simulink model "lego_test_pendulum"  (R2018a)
settings: Solver=VariableStepAuto  StartTime=0.0  StopTime=3  RelTol=1e-3
model workspace: external: MATLAB File (data not in the file)
undefined symbols (not defined in the file): cm, deg, kg, m, mm, N, rad, s, smiData, X, Y, Z
libraries: sm_lib x60, nesl_utility x3, simulink_extras x2
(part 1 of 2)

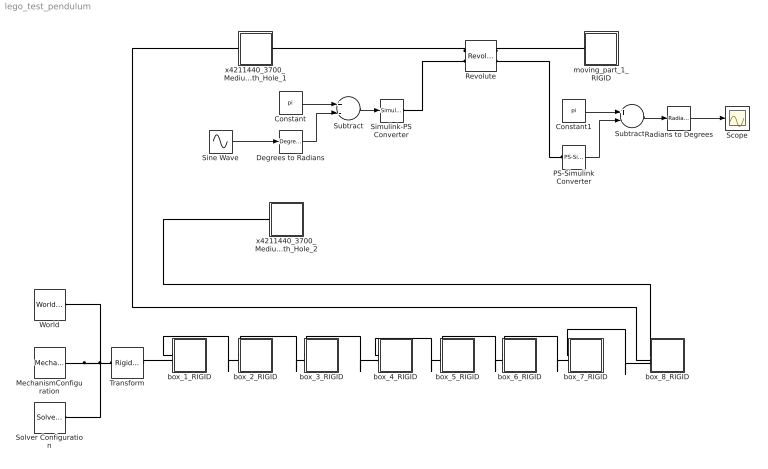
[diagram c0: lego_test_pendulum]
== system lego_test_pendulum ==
  Constant : Constant  Value=pi
  Constant1 : Constant  Value=pi
  Degrees to Radians : simulink_extras/Transformations/Degrees to Radians
  MechanismConfiguration : sm_lib/Utilities/Mechanism Configuration  UniformGravity=Constant  GravityVector=[0 -9.80665 0]  GravityUnits=m/s^2  LinearizationDelta=0.001
  PS-Simulink Converter : nesl_utility/PS-Simulink Converter  PhysicalDomain=network_engine_domain  SubClassName=ps_output  LeftPortType=input  RightPortType=output  PseudoPeriodic=off  Frequencies=[]  Unit=rad  AffineConversion=off
  Radians to Degrees : simulink_extras/Transformations/Radians to Degrees
  Revolute : sm_lib/Joints/Revolute Joint  SenseConstraintForce=off  SenseConstraintForceX=off  SenseConstraintForceY=off  SenseConstraintForceZ=off  SenseConstraintTorque=off  SenseConstraintTorqueX=off  SenseConstraintTorqueY=off  SenseConstraintTorqueZ=off  SenseTotalForce=off  SenseTotalForceX=off  SenseTotalForceY=off  SenseTotalForceZ=off  SenseTotalTorque=off  SenseTotalTorqueX=off  SenseTotalTorqueY=off  SenseTotalTorqueZ=off  CompositeWrenchDir=FollowerOnBase  CompositeWrenchFrame=BaseFrame  EquilibriumPosition=0  EquilibriumPositionUnits=rad  SpringStiffness=0  SpringStiffnessUnits=N*m/rad  DampingCoefficient=0  DampingCoefficientUnits=N*m/(rad/s)  TorqueActuationMode=ComputedTorque  MotionActuationMode=InputMotion  SensePosition=on  SenseVelocity=off  SenseAcceleration=off  SenseTorqueForce=off  PositionTargetSpecify=on  PositionTargetPriority=Low  PositionTargetValue=pi  PositionTargetValueUnits=rad  VelocityTargetSpecify=off  VelocityTargetPriority=High  VelocityTargetValue=0  VelocityTargetValueUnits=deg/s
  Scope : Scope
  Simulink-PS Converter : nesl_utility/Simulink-PS Converter  PhysicalDomain=network_engine_domain  SubClassName=ps_input  LeftPortType=input  RightPortType=output  PseudoPeriodic=off  Frequencies=[]  NoiseDistribution=none  NoiseParameters=[]  Unit=rad  AffineConversion=off  FilteringAndDerivatives=filter  SimscapeFilterOrder=2  InputFilterTimeConstant=0.001  UdotUserProvided=0
  Sine Wave : Sin  Amplitude=30  Frequency=2*pi  SampleTime=0
  Solver Configuration : nesl_utility/Solver Configuration  PhysicalDomain=network_engine_domain  SubClassName=solver  LeftPortType=input  RightPortType=generic  Tones=[]  Harmonics=[]  SimulateNoise=off  Profile=off  UseLocalSampling=off  EnableSwitchedLinearOptims=on  FrequencyDomain=off  UseCCode=off  RelTol=0.001  AbsTol=1e-06  MinStep=1e-09  ToWorkspace=off  RevertToSquareIcSolve=off  NumHomotopyIterations=100  PhasorMode=off  PhasorModeNumHarmonics=1  DoDC=off  ResidualTolerance=1e-09  UseLocalSolver=off  LocalSolverChoice=NE_BACKWARD_EULER_ADVANCER  LocalSolverSampleTime=0.001  DoFixedCost=off  MaxNonlinIter=3  MaxModeIter=2  LinearAlgebra=Sparse  EquationFormulation=NE_TIME_EF  DelaysMemoryBudget=1024  AutomaticFiltering=on  FilteringTimeConstant=0.001
  Subtract : Sum  Inputs=+-
  Subtract1 : Sum  Inputs=+-
  Transform : sm_lib/Frames and Transforms/Rigid Transform  TranslationMethod=Cartesian  TranslationStandardOffset=0  TranslationLengthUnit=mm  TranslationStandardAxis=+Z  TranslationCartesianOffset=smiData.RigidTransform(26).translation  TranslationROffset=0  TranslationROffsetUnits=m  TranslationZOffset=0  TranslationZOffsetUnits=m  TranslationThetaOffset=0  TranslationThetaOffsetUnits=deg  RotationMethod=ArbitraryAxis  RotationAngleUnits=rad  RotationStandardAxis=+Z  RotationAngle=smiData.RigidTransform(26).angle  RotationArbitraryAxis=smiData.RigidTransform(26).axis  FollAlignAxisA=+X  BaseAlignAxisA=+Y  FollAlignAxisB=+Y  BaseAlignAxisB=+Z  RotationSequenceAxes=FollowerAxes  RotationSequence=XYX  RotationSequenceAngles=[0 0 0]  RotationSequenceAnglesUnits=deg  RotationMatrix=[1 0 0; 0 1 0; 0 0 1]
  World : sm_lib/Frames and Transforms/World Frame
  box_1_RIGID : Subsystem
  box_2_RIGID : Subsystem
  box_3_RIGID : Subsystem
  box_4_RIGID : Subsystem
  box_5_RIGID : Subsystem
  box_6_RIGID : Subsystem
  box_7_RIGID : Subsystem
  box_8_RIGID : Subsystem
  moving_part_1_RIGID : Subsystem
  x4211440_3700_Medium_Stone_Grey_Technic_Brick_1_x_2_with_Hole_1 : Subsystem
  x4211440_3700_Medium_Stone_Grey_Technic_Brick_1_x_2_with_Hole_2 : Subsystem
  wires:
  Radians to Degrees/1 -> Scope/1
  Constant/1 -> Subtract/1
  Subtract/1 -> Simulink-PS Converter/1
  Constant1/1 -> Subtract1/1
  PS-Simulink Converter/1 -> Subtract1/2
  Subtract1/1 -> Radians to Degrees/1
  Degrees to Radians/1 -> Subtract/2
  Sine Wave/1 -> Degrees to Radians/1
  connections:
  Transform/LConn1 -- MechanismConfiguration/RConn1 -- Solver Configuration/RConn1 -- World/RConn1
  Revolute/LConn1 -- x4211440_3700_Medium_Stone_Grey_Technic_Brick_1_x_2_with_Hole_1/RConn1
  box_8_RIGID/LConn2 -- x4211440_3700_Medium_Stone_Grey_Technic_Brick_1_x_2_with_Hole_1/LConn1
  box_8_RIGID/LConn1 -- x4211440_3700_Medium_Stone_Grey_Technic_Brick_1_x_2_with_Hole_2/LConn1
  Transform/RConn1 -- box_1_RIGID/LConn2
  Revolute/RConn1 -- moving_part_1_RIGID/LConn1
  box_1_RIGID/LConn1 -- box_2_RIGID/LConn2
  box_2_RIGID/LConn1 -- box_3_RIGID/LConn2
  box_3_RIGID/LConn1 -- box_4_RIGID/LConn2
  box_4_RIGID/LConn1 -- box_5_RIGID/LConn2
  box_5_RIGID/LConn1 -- box_6_RIGID/LConn2
  box_6_RIGID/LConn1 -- box_7_RIGID/LConn2
  box_7_RIGID/LConn1 -- box_8_RIGID/LConn3
  PS-Simulink Converter/LConn1 -- Revolute/RConn2
  Simulink-PS Converter/RConn1 -- Revolute/LConn2

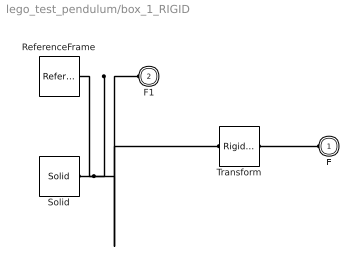
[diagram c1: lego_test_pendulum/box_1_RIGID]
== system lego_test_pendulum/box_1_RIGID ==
  ReferenceFrame : sm_lib/Frames and Transforms/Reference Frame
  Solid : sm_lib/Body Elements/Solid  InertiaType=Custom  Mass=smiData.Solid(1).mass  MassUnits=kg  CenterOfMass=smiData.Solid(1).CoM  CenterOfMassUnits=mm  MomentsOfInertia=smiData.Solid(1).MoI  MomentsOfInertiaUnits=kg*mm^2  ProductsOfInertia=smiData.Solid(1).PoI  ProductsOfInertiaUnits=kg*mm^2  DensityBased=on  Density=1000  DensityUnits=kg/m^3  DoExposeReferenceFrame=on  SerializedFrames=<Frames/>  GraphicType=FromGeometry  MarkerShape=Sphere  MarkerSize=10  GraphicVisPropType=SimpleVisualProperties  GraphicDiffuseColor=smiData.Solid(1).color  GraphicSpecularColor=[0.5 0.5 0.5 1.0]  GraphicAmbientColor=[0.15 0.15 0.15 1.0]  GraphicEmissiveColor=[0.0 0.0 0.0 1.0]  GraphicShininess=75  GraphicOpacity=smiData.Solid(1).opacity  GeometryShape=FromFile  RectangleSize=[1 1]  RectangleSizeUnits=m  BrickDimensions=[1 1 1]  BrickDimensionUnits=m  CylinderRadius=1  CylinderRadiusUnits=m  CylinderLength=1  CylinderLengthUnits=m  SphereRadius=1  SphereRadiusUnits=m  EllipsoidRadii=[1 1 1]  EllipsoidRadiiUnits=m  ExtrusionCrossSection=[1 1; -1 1; -1 -1; 1 -1]  ExtrusionCrossSectionUnits=m  ExtrusionLength=1  ExtrusionLengthUnits=m  PolygonNumSides=3  PolygonOuterRadius=1  PolygonOuterRadiusUnits=m  ExtGeomFileType=STEP  ExtGeomFileName=box_Predeterminado_sldprt.STEP  ExtGeomFileUnits=m  RevolutionCrossSection=[1 1; 1 -1; 2 -1; 2 1]  RevolutionCrossSectionUnits=m  RevolutionExtent=Full  RevolutionAngle=180  RevolutionAngleUnits=deg
  Transform : sm_lib/Frames and Transforms/Rigid Transform  TranslationMethod=Cartesian  TranslationStandardOffset=0  TranslationLengthUnit=mm  TranslationStandardAxis=+Z  TranslationCartesianOffset=smiData.RigidTransform(3).translation  TranslationROffset=0  TranslationROffsetUnits=m  TranslationZOffset=0  TranslationZOffsetUnits=m  TranslationThetaOffset=0  TranslationThetaOffsetUnits=deg  RotationMethod=ArbitraryAxis  RotationAngleUnits=rad  RotationStandardAxis=+Z  RotationAngle=smiData.RigidTransform(3).angle  RotationArbitraryAxis=smiData.RigidTransform(3).axis  FollAlignAxisA=+X  BaseAlignAxisA=+Y  FollAlignAxisB=+Y  BaseAlignAxisB=+Z  RotationSequenceAxes=FollowerAxes  RotationSequence=XYX  RotationSequenceAngles=[0 0 0]  RotationSequenceAnglesUnits=deg  RotationMatrix=[1 0 0; 0 1 0; 0 0 1]
  F : PMIOPort  Side=Left
  F1 : PMIOPort  Port=2  Side=Left
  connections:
  Solid/RConn1 -- ReferenceFrame/RConn1 -- Transform/LConn1 -- F1/RConn1
  Transform/RConn1 -- F/RConn1

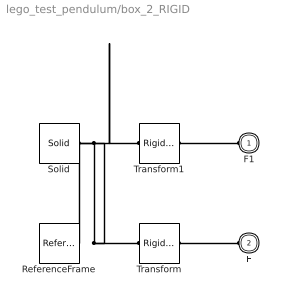
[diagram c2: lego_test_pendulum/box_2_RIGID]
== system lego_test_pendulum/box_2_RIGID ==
  ReferenceFrame : sm_lib/Frames and Transforms/Reference Frame
  Solid : sm_lib/Body Elements/Solid  InertiaType=Custom  Mass=smiData.Solid(1).mass  MassUnits=kg  CenterOfMass=smiData.Solid(1).CoM  CenterOfMassUnits=mm  MomentsOfInertia=smiData.Solid(1).MoI  MomentsOfInertiaUnits=kg*mm^2  ProductsOfInertia=smiData.Solid(1).PoI  ProductsOfInertiaUnits=kg*mm^2  DensityBased=on  Density=1000  DensityUnits=kg/m^3  DoExposeReferenceFrame=on  SerializedFrames=<Frames/>  GraphicType=FromGeometry  MarkerShape=Sphere  MarkerSize=10  GraphicVisPropType=SimpleVisualProperties  GraphicDiffuseColor=smiData.Solid(1).color  GraphicSpecularColor=[0.5 0.5 0.5 1.0]  GraphicAmbientColor=[0.15 0.15 0.15 1.0]  GraphicEmissiveColor=[0.0 0.0 0.0 1.0]  GraphicShininess=75  GraphicOpacity=smiData.Solid(1).opacity  GeometryShape=FromFile  RectangleSize=[1 1]  RectangleSizeUnits=m  BrickDimensions=[1 1 1]  BrickDimensionUnits=m  CylinderRadius=1  CylinderRadiusUnits=m  CylinderLength=1  CylinderLengthUnits=m  SphereRadius=1  SphereRadiusUnits=m  EllipsoidRadii=[1 1 1]  EllipsoidRadiiUnits=m  ExtrusionCrossSection=[1 1; -1 1; -1 -1; 1 -1]  ExtrusionCrossSectionUnits=m  ExtrusionLength=1  ExtrusionLengthUnits=m  PolygonNumSides=3  PolygonOuterRadius=1  PolygonOuterRadiusUnits=m  ExtGeomFileType=STEP  ExtGeomFileName=box_Predeterminado_sldprt.STEP  ExtGeomFileUnits=m  RevolutionCrossSection=[1 1; 1 -1; 2 -1; 2 1]  RevolutionCrossSectionUnits=m  RevolutionExtent=Full  RevolutionAngle=180  RevolutionAngleUnits=deg
  Transform : sm_lib/Frames and Transforms/Rigid Transform  TranslationMethod=Cartesian  TranslationStandardOffset=0  TranslationLengthUnit=mm  TranslationStandardAxis=+Z  TranslationCartesianOffset=smiData.RigidTransform(4).translation  TranslationROffset=0  TranslationROffsetUnits=m  TranslationZOffset=0  TranslationZOffsetUnits=m  TranslationThetaOffset=0  TranslationThetaOffsetUnits=deg  RotationMethod=ArbitraryAxis  RotationAngleUnits=rad  RotationStandardAxis=+Z  RotationAngle=smiData.RigidTransform(4).angle  RotationArbitraryAxis=smiData.RigidTransform(4).axis  FollAlignAxisA=+X  BaseAlignAxisA=+Y  FollAlignAxisB=+Y  BaseAlignAxisB=+Z  RotationSequenceAxes=FollowerAxes  RotationSequence=XYX  RotationSequenceAngles=[0 0 0]  RotationSequenceAnglesUnits=deg  RotationMatrix=[1 0 0; 0 1 0; 0 0 1]
  Transform1 : sm_lib/Frames and Transforms/Rigid Transform  TranslationMethod=Cartesian  TranslationStandardOffset=0  TranslationLengthUnit=mm  TranslationStandardAxis=+Z  TranslationCartesianOffset=smiData.RigidTransform(5).translation  TranslationROffset=0  TranslationROffsetUnits=m  TranslationZOffset=0  TranslationZOffsetUnits=m  TranslationThetaOffset=0  TranslationThetaOffsetUnits=deg  RotationMethod=ArbitraryAxis  RotationAngleUnits=rad  RotationStandardAxis=+Z  RotationAngle=smiData.RigidTransform(5).angle  RotationArbitraryAxis=smiData.RigidTransform(5).axis  FollAlignAxisA=+X  BaseAlignAxisA=+Y  FollAlignAxisB=+Y  BaseAlignAxisB=+Z  RotationSequenceAxes=FollowerAxes  RotationSequence=XYX  RotationSequenceAngles=[0 0 0]  RotationSequenceAnglesUnits=deg  RotationMatrix=[1 0 0; 0 1 0; 0 0 1]
  F1 : PMIOPort  Side=Left
  F : PMIOPort  Port=2  Side=Left
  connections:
  Solid/RConn1 -- ReferenceFrame/RConn1 -- Transform/LConn1 -- Transform1/LConn1
  Transform/RConn1 -- F/RConn1
  Transform1/RConn1 -- F1/RConn1

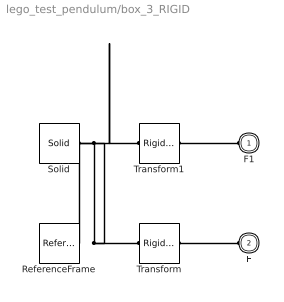
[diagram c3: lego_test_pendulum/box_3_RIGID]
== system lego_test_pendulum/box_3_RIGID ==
  ReferenceFrame : sm_lib/Frames and Transforms/Reference Frame
  Solid : sm_lib/Body Elements/Solid  InertiaType=Custom  Mass=smiData.Solid(1).mass  MassUnits=kg  CenterOfMass=smiData.Solid(1).CoM  CenterOfMassUnits=mm  MomentsOfInertia=smiData.Solid(1).MoI  MomentsOfInertiaUnits=kg*mm^2  ProductsOfInertia=smiData.Solid(1).PoI  ProductsOfInertiaUnits=kg*mm^2  DensityBased=on  Density=1000  DensityUnits=kg/m^3  DoExposeReferenceFrame=on  SerializedFrames=<Frames/>  GraphicType=FromGeometry  MarkerShape=Sphere  MarkerSize=10  GraphicVisPropType=SimpleVisualProperties  GraphicDiffuseColor=smiData.Solid(1).color  GraphicSpecularColor=[0.5 0.5 0.5 1.0]  GraphicAmbientColor=[0.15 0.15 0.15 1.0]  GraphicEmissiveColor=[0.0 0.0 0.0 1.0]  GraphicShininess=75  GraphicOpacity=smiData.Solid(1).opacity  GeometryShape=FromFile  RectangleSize=[1 1]  RectangleSizeUnits=m  BrickDimensions=[1 1 1]  BrickDimensionUnits=m  CylinderRadius=1  CylinderRadiusUnits=m  CylinderLength=1  CylinderLengthUnits=m  SphereRadius=1  SphereRadiusUnits=m  EllipsoidRadii=[1 1 1]  EllipsoidRadiiUnits=m  ExtrusionCrossSection=[1 1; -1 1; -1 -1; 1 -1]  ExtrusionCrossSectionUnits=m  ExtrusionLength=1  ExtrusionLengthUnits=m  PolygonNumSides=3  PolygonOuterRadius=1  PolygonOuterRadiusUnits=m  ExtGeomFileType=STEP  ExtGeomFileName=box_Predeterminado_sldprt.STEP  ExtGeomFileUnits=m  RevolutionCrossSection=[1 1; 1 -1; 2 -1; 2 1]  RevolutionCrossSectionUnits=m  RevolutionExtent=Full  RevolutionAngle=180  RevolutionAngleUnits=deg
  Transform : sm_lib/Frames and Transforms/Rigid Transform  TranslationMethod=Cartesian  TranslationStandardOffset=0  TranslationLengthUnit=mm  TranslationStandardAxis=+Z  TranslationCartesianOffset=smiData.RigidTransform(6).translation  TranslationROffset=0  TranslationROffsetUnits=m  TranslationZOffset=0  TranslationZOffsetUnits=m  TranslationThetaOffset=0  TranslationThetaOffsetUnits=deg  RotationMethod=ArbitraryAxis  RotationAngleUnits=rad  RotationStandardAxis=+Z  RotationAngle=smiData.RigidTransform(6).angle  RotationArbitraryAxis=smiData.RigidTransform(6).axis  FollAlignAxisA=+X  BaseAlignAxisA=+Y  FollAlignAxisB=+Y  BaseAlignAxisB=+Z  RotationSequenceAxes=FollowerAxes  RotationSequence=XYX  RotationSequenceAngles=[0 0 0]  RotationSequenceAnglesUnits=deg  RotationMatrix=[1 0 0; 0 1 0; 0 0 1]
  Transform1 : sm_lib/Frames and Transforms/Rigid Transform  TranslationMethod=Cartesian  TranslationStandardOffset=0  TranslationLengthUnit=mm  TranslationStandardAxis=+Z  TranslationCartesianOffset=smiData.RigidTransform(7).translation  TranslationROffset=0  TranslationROffsetUnits=m  TranslationZOffset=0  TranslationZOffsetUnits=m  TranslationThetaOffset=0  TranslationThetaOffsetUnits=deg  RotationMethod=ArbitraryAxis  RotationAngleUnits=rad  RotationStandardAxis=+Z  RotationAngle=smiData.RigidTransform(7).angle  RotationArbitraryAxis=smiData.RigidTransform(7).axis  FollAlignAxisA=+X  BaseAlignAxisA=+Y  FollAlignAxisB=+Y  BaseAlignAxisB=+Z  RotationSequenceAxes=FollowerAxes  RotationSequence=XYX  RotationSequenceAngles=[0 0 0]  RotationSequenceAnglesUnits=deg  RotationMatrix=[1 0 0; 0 1 0; 0 0 1]
  F1 : PMIOPort  Side=Left
  F : PMIOPort  Port=2  Side=Left
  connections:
  Solid/RConn1 -- ReferenceFrame/RConn1 -- Transform/LConn1 -- Transform1/LConn1
  Transform/RConn1 -- F/RConn1
  Transform1/RConn1 -- F1/RConn1

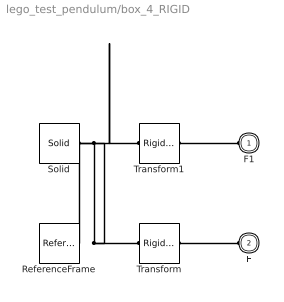
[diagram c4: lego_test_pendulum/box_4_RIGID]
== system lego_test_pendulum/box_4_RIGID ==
  ReferenceFrame : sm_lib/Frames and Transforms/Reference Frame
  Solid : sm_lib/Body Elements/Solid  InertiaType=Custom  Mass=smiData.Solid(1).mass  MassUnits=kg  CenterOfMass=smiData.Solid(1).CoM  CenterOfMassUnits=mm  MomentsOfInertia=smiData.Solid(1).MoI  MomentsOfInertiaUnits=kg*mm^2  ProductsOfInertia=smiData.Solid(1).PoI  ProductsOfInertiaUnits=kg*mm^2  DensityBased=on  Density=1000  DensityUnits=kg/m^3  DoExposeReferenceFrame=on  SerializedFrames=<Frames/>  GraphicType=FromGeometry  MarkerShape=Sphere  MarkerSize=10  GraphicVisPropType=SimpleVisualProperties  GraphicDiffuseColor=smiData.Solid(1).color  GraphicSpecularColor=[0.5 0.5 0.5 1.0]  GraphicAmbientColor=[0.15 0.15 0.15 1.0]  GraphicEmissiveColor=[0.0 0.0 0.0 1.0]  GraphicShininess=75  GraphicOpacity=smiData.Solid(1).opacity  GeometryShape=FromFile  RectangleSize=[1 1]  RectangleSizeUnits=m  BrickDimensions=[1 1 1]  BrickDimensionUnits=m  CylinderRadius=1  CylinderRadiusUnits=m  CylinderLength=1  CylinderLengthUnits=m  SphereRadius=1  SphereRadiusUnits=m  EllipsoidRadii=[1 1 1]  EllipsoidRadiiUnits=m  ExtrusionCrossSection=[1 1; -1 1; -1 -1; 1 -1]  ExtrusionCrossSectionUnits=m  ExtrusionLength=1  ExtrusionLengthUnits=m  PolygonNumSides=3  PolygonOuterRadius=1  PolygonOuterRadiusUnits=m  ExtGeomFileType=STEP  ExtGeomFileName=box_Predeterminado_sldprt.STEP  ExtGeomFileUnits=m  RevolutionCrossSection=[1 1; 1 -1; 2 -1; 2 1]  RevolutionCrossSectionUnits=m  RevolutionExtent=Full  RevolutionAngle=180  RevolutionAngleUnits=deg
  Transform : sm_lib/Frames and Transforms/Rigid Transform  TranslationMethod=Cartesian  TranslationStandardOffset=0  TranslationLengthUnit=mm  TranslationStandardAxis=+Z  TranslationCartesianOffset=smiData.RigidTransform(8).translation  TranslationROffset=0  TranslationROffsetUnits=m  TranslationZOffset=0  TranslationZOffsetUnits=m  TranslationThetaOffset=0  TranslationThetaOffsetUnits=deg  RotationMethod=ArbitraryAxis  RotationAngleUnits=rad  RotationStandardAxis=+Z  RotationAngle=smiData.RigidTransform(8).angle  RotationArbitraryAxis=smiData.RigidTransform(8).axis  FollAlignAxisA=+X  BaseAlignAxisA=+Y  FollAlignAxisB=+Y  BaseAlignAxisB=+Z  RotationSequenceAxes=FollowerAxes  RotationSequence=XYX  RotationSequenceAngles=[0 0 0]  RotationSequenceAnglesUnits=deg  RotationMatrix=[1 0 0; 0 1 0; 0 0 1]
  Transform1 : sm_lib/Frames and Transforms/Rigid Transform  TranslationMethod=Cartesian  TranslationStandardOffset=0  TranslationLengthUnit=mm  TranslationStandardAxis=+Z  TranslationCartesianOffset=smiData.RigidTransform(9).translation  TranslationROffset=0  TranslationROffsetUnits=m  TranslationZOffset=0  TranslationZOffsetUnits=m  TranslationThetaOffset=0  TranslationThetaOffsetUnits=deg  RotationMethod=ArbitraryAxis  RotationAngleUnits=rad  RotationStandardAxis=+Z  RotationAngle=smiData.RigidTransform(9).angle  RotationArbitraryAxis=smiData.RigidTransform(9).axis  FollAlignAxisA=+X  BaseAlignAxisA=+Y  FollAlignAxisB=+Y  BaseAlignAxisB=+Z  RotationSequenceAxes=FollowerAxes  RotationSequence=XYX  RotationSequenceAngles=[0 0 0]  RotationSequenceAnglesUnits=deg  RotationMatrix=[1 0 0; 0 1 0; 0 0 1]
  F1 : PMIOPort  Side=Left
  F : PMIOPort  Port=2  Side=Left
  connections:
  Solid/RConn1 -- ReferenceFrame/RConn1 -- Transform/LConn1 -- Transform1/LConn1
  Transform/RConn1 -- F/RConn1
  Transform1/RConn1 -- F1/RConn1

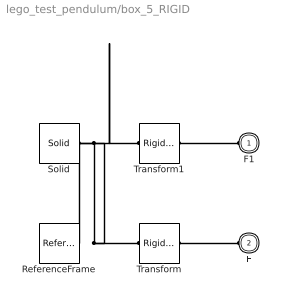
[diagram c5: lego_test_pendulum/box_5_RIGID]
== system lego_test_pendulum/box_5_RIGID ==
  ReferenceFrame : sm_lib/Frames and Transforms/Reference Frame
  Solid : sm_lib/Body Elements/Solid  InertiaType=Custom  Mass=smiData.Solid(1).mass  MassUnits=kg  CenterOfMass=smiData.Solid(1).CoM  CenterOfMassUnits=mm  MomentsOfInertia=smiData.Solid(1).MoI  MomentsOfInertiaUnits=kg*mm^2  ProductsOfInertia=smiData.Solid(1).PoI  ProductsOfInertiaUnits=kg*mm^2  DensityBased=on  Density=1000  DensityUnits=kg/m^3  DoExposeReferenceFrame=on  SerializedFrames=<Frames/>  GraphicType=FromGeometry  MarkerShape=Sphere  MarkerSize=10  GraphicVisPropType=SimpleVisualProperties  GraphicDiffuseColor=smiData.Solid(1).color  GraphicSpecularColor=[0.5 0.5 0.5 1.0]  GraphicAmbientColor=[0.15 0.15 0.15 1.0]  GraphicEmissiveColor=[0.0 0.0 0.0 1.0]  GraphicShininess=75  GraphicOpacity=smiData.Solid(1).opacity  GeometryShape=FromFile  RectangleSize=[1 1]  RectangleSizeUnits=m  BrickDimensions=[1 1 1]  BrickDimensionUnits=m  CylinderRadius=1  CylinderRadiusUnits=m  CylinderLength=1  CylinderLengthUnits=m  SphereRadius=1  SphereRadiusUnits=m  EllipsoidRadii=[1 1 1]  EllipsoidRadiiUnits=m  ExtrusionCrossSection=[1 1; -1 1; -1 -1; 1 -1]  ExtrusionCrossSectionUnits=m  ExtrusionLength=1  ExtrusionLengthUnits=m  PolygonNumSides=3  PolygonOuterRadius=1  PolygonOuterRadiusUnits=m  ExtGeomFileType=STEP  ExtGeomFileName=box_Predeterminado_sldprt.STEP  ExtGeomFileUnits=m  RevolutionCrossSection=[1 1; 1 -1; 2 -1; 2 1]  RevolutionCrossSectionUnits=m  RevolutionExtent=Full  RevolutionAngle=180  RevolutionAngleUnits=deg
  Transform : sm_lib/Frames and Transforms/Rigid Transform  TranslationMethod=Cartesian  TranslationStandardOffset=0  TranslationLengthUnit=mm  TranslationStandardAxis=+Z  TranslationCartesianOffset=smiData.RigidTransform(10).translation  TranslationROffset=0  TranslationROffsetUnits=m  TranslationZOffset=0  TranslationZOffsetUnits=m  TranslationThetaOffset=0  TranslationThetaOffsetUnits=deg  RotationMethod=ArbitraryAxis  RotationAngleUnits=rad  RotationStandardAxis=+Z  RotationAngle=smiData.RigidTransform(10).angle  RotationArbitraryAxis=smiData.RigidTransform(10).axis  FollAlignAxisA=+X  BaseAlignAxisA=+Y  FollAlignAxisB=+Y  BaseAlignAxisB=+Z  RotationSequenceAxes=FollowerAxes  RotationSequence=XYX  RotationSequenceAngles=[0 0 0]  RotationSequenceAnglesUnits=deg  RotationMatrix=[1 0 0; 0 1 0; 0 0 1]
  Transform1 : sm_lib/Frames and Transforms/Rigid Transform  TranslationMethod=Cartesian  TranslationStandardOffset=0  TranslationLengthUnit=mm  TranslationStandardAxis=+Z  TranslationCartesianOffset=smiData.RigidTransform(11).translation  TranslationROffset=0  TranslationROffsetUnits=m  TranslationZOffset=0  TranslationZOffsetUnits=m  TranslationThetaOffset=0  TranslationThetaOffsetUnits=deg  RotationMethod=ArbitraryAxis  RotationAngleUnits=rad  RotationStandardAxis=+Z  RotationAngle=smiData.RigidTransform(11).angle  RotationArbitraryAxis=smiData.RigidTransform(11).axis  FollAlignAxisA=+X  BaseAlignAxisA=+Y  FollAlignAxisB=+Y  BaseAlignAxisB=+Z  RotationSequenceAxes=FollowerAxes  RotationSequence=XYX  RotationSequenceAngles=[0 0 0]  RotationSequenceAnglesUnits=deg  RotationMatrix=[1 0 0; 0 1 0; 0 0 1]
  F1 : PMIOPort  Side=Left
  F : PMIOPort  Port=2  Side=Left
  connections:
  Solid/RConn1 -- ReferenceFrame/RConn1 -- Transform/LConn1 -- Transform1/LConn1
  Transform/RConn1 -- F/RConn1
  Transform1/RConn1 -- F1/RConn1

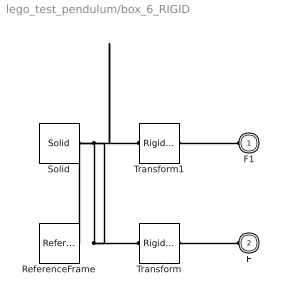
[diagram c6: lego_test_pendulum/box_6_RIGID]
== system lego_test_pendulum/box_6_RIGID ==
  ReferenceFrame : sm_lib/Frames and Transforms/Reference Frame
  Solid : sm_lib/Body Elements/Solid  InertiaType=Custom  Mass=smiData.Solid(1).mass  MassUnits=kg  CenterOfMass=smiData.Solid(1).CoM  CenterOfMassUnits=mm  MomentsOfInertia=smiData.Solid(1).MoI  MomentsOfInertiaUnits=kg*mm^2  ProductsOfInertia=smiData.Solid(1).PoI  ProductsOfInertiaUnits=kg*mm^2  DensityBased=on  Density=1000  DensityUnits=kg/m^3  DoExposeReferenceFrame=on  SerializedFrames=<Frames/>  GraphicType=FromGeometry  MarkerShape=Sphere  MarkerSize=10  GraphicVisPropType=SimpleVisualProperties  GraphicDiffuseColor=smiData.Solid(1).color  GraphicSpecularColor=[0.5 0.5 0.5 1.0]  GraphicAmbientColor=[0.15 0.15 0.15 1.0]  GraphicEmissiveColor=[0.0 0.0 0.0 1.0]  GraphicShininess=75  GraphicOpacity=smiData.Solid(1).opacity  GeometryShape=FromFile  RectangleSize=[1 1]  RectangleSizeUnits=m  BrickDimensions=[1 1 1]  BrickDimensionUnits=m  CylinderRadius=1  CylinderRadiusUnits=m  CylinderLength=1  CylinderLengthUnits=m  SphereRadius=1  SphereRadiusUnits=m  EllipsoidRadii=[1 1 1]  EllipsoidRadiiUnits=m  ExtrusionCrossSection=[1 1; -1 1; -1 -1; 1 -1]  ExtrusionCrossSectionUnits=m  ExtrusionLength=1  ExtrusionLengthUnits=m  PolygonNumSides=3  PolygonOuterRadius=1  PolygonOuterRadiusUnits=m  ExtGeomFileType=STEP  ExtGeomFileName=box_Predeterminado_sldprt.STEP  ExtGeomFileUnits=m  RevolutionCrossSection=[1 1; 1 -1; 2 -1; 2 1]  RevolutionCrossSectionUnits=m  RevolutionExtent=Full  RevolutionAngle=180  RevolutionAngleUnits=deg
  Transform : sm_lib/Frames and Transforms/Rigid Transform  TranslationMethod=Cartesian  TranslationStandardOffset=0  TranslationLengthUnit=mm  TranslationStandardAxis=+Z  TranslationCartesianOffset=smiData.RigidTransform(12).translation  TranslationROffset=0  TranslationROffsetUnits=m  TranslationZOffset=0  TranslationZOffsetUnits=m  TranslationThetaOffset=0  TranslationThetaOffsetUnits=deg  RotationMethod=ArbitraryAxis  RotationAngleUnits=rad  RotationStandardAxis=+Z  RotationAngle=smiData.RigidTransform(12).angle  RotationArbitraryAxis=smiData.RigidTransform(12).axis  FollAlignAxisA=+X  BaseAlignAxisA=+Y  FollAlignAxisB=+Y  BaseAlignAxisB=+Z  RotationSequenceAxes=FollowerAxes  RotationSequence=XYX  RotationSequenceAngles=[0 0 0]  RotationSequenceAnglesUnits=deg  RotationMatrix=[1 0 0; 0 1 0; 0 0 1]
  Transform1 : sm_lib/Frames and Transforms/Rigid Transform  TranslationMethod=Cartesian  TranslationStandardOffset=0  TranslationLengthUnit=mm  TranslationStandardAxis=+Z  TranslationCartesianOffset=smiData.RigidTransform(13).translation  TranslationROffset=0  TranslationROffsetUnits=m  TranslationZOffset=0  TranslationZOffsetUnits=m  TranslationThetaOffset=0  TranslationThetaOffsetUnits=deg  RotationMethod=ArbitraryAxis  RotationAngleUnits=rad  RotationStandardAxis=+Z  RotationAngle=smiData.RigidTransform(13).angle  RotationArbitraryAxis=smiData.RigidTransform(13).axis  FollAlignAxisA=+X  BaseAlignAxisA=+Y  FollAlignAxisB=+Y  BaseAlignAxisB=+Z  RotationSequenceAxes=FollowerAxes  RotationSequence=XYX  RotationSequenceAngles=[0 0 0]  RotationSequenceAnglesUnits=deg  RotationMatrix=[1 0 0; 0 1 0; 0 0 1]
  F1 : PMIOPort  Side=Left
  F : PMIOPort  Port=2  Side=Left
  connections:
  Solid/RConn1 -- ReferenceFrame/RConn1 -- Transform/LConn1 -- Transform1/LConn1
  Transform/RConn1 -- F/RConn1
  Transform1/RConn1 -- F1/RConn1

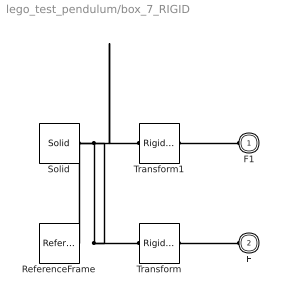
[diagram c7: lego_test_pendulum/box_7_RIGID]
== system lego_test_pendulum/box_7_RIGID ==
  ReferenceFrame : sm_lib/Frames and Transforms/Reference Frame
  Solid : sm_lib/Body Elements/Solid  InertiaType=Custom  Mass=smiData.Solid(1).mass  MassUnits=kg  CenterOfMass=smiData.Solid(1).CoM  CenterOfMassUnits=mm  MomentsOfInertia=smiData.Solid(1).MoI  MomentsOfInertiaUnits=kg*mm^2  ProductsOfInertia=smiData.Solid(1).PoI  ProductsOfInertiaUnits=kg*mm^2  DensityBased=on  Density=1000  DensityUnits=kg/m^3  DoExposeReferenceFrame=on  SerializedFrames=<Frames/>  GraphicType=FromGeometry  MarkerShape=Sphere  MarkerSize=10  GraphicVisPropType=SimpleVisualProperties  GraphicDiffuseColor=smiData.Solid(1).color  GraphicSpecularColor=[0.5 0.5 0.5 1.0]  GraphicAmbientColor=[0.15 0.15 0.15 1.0]  GraphicEmissiveColor=[0.0 0.0 0.0 1.0]  GraphicShininess=75  GraphicOpacity=smiData.Solid(1).opacity  GeometryShape=FromFile  RectangleSize=[1 1]  RectangleSizeUnits=m  BrickDimensions=[1 1 1]  BrickDimensionUnits=m  CylinderRadius=1  CylinderRadiusUnits=m  CylinderLength=1  CylinderLengthUnits=m  SphereRadius=1  SphereRadiusUnits=m  EllipsoidRadii=[1 1 1]  EllipsoidRadiiUnits=m  ExtrusionCrossSection=[1 1; -1 1; -1 -1; 1 -1]  ExtrusionCrossSectionUnits=m  ExtrusionLength=1  ExtrusionLengthUnits=m  PolygonNumSides=3  PolygonOuterRadius=1  PolygonOuterRadiusUnits=m  ExtGeomFileType=STEP  ExtGeomFileName=box_Predeterminado_sldprt.STEP  ExtGeomFileUnits=m  RevolutionCrossSection=[1 1; 1 -1; 2 -1; 2 1]  RevolutionCrossSectionUnits=m  RevolutionExtent=Full  RevolutionAngle=180  RevolutionAngleUnits=deg
  Transform : sm_lib/Frames and Transforms/Rigid Transform  TranslationMethod=Cartesian  TranslationStandardOffset=0  TranslationLengthUnit=mm  TranslationStandardAxis=+Z  TranslationCartesianOffset=smiData.RigidTransform(14).translation  TranslationROffset=0  TranslationROffsetUnits=m  TranslationZOffset=0  TranslationZOffsetUnits=m  TranslationThetaOffset=0  TranslationThetaOffsetUnits=deg  RotationMethod=ArbitraryAxis  RotationAngleUnits=rad  RotationStandardAxis=+Z  RotationAngle=smiData.RigidTransform(14).angle  RotationArbitraryAxis=smiData.RigidTransform(14).axis  FollAlignAxisA=+X  BaseAlignAxisA=+Y  FollAlignAxisB=+Y  BaseAlignAxisB=+Z  RotationSequenceAxes=FollowerAxes  RotationSequence=XYX  RotationSequenceAngles=[0 0 0]  RotationSequenceAnglesUnits=deg  RotationMatrix=[1 0 0; 0 1 0; 0 0 1]
  Transform1 : sm_lib/Frames and Transforms/Rigid Transform  TranslationMethod=Cartesian  TranslationStandardOffset=0  TranslationLengthUnit=mm  TranslationStandardAxis=+Z  TranslationCartesianOffset=smiData.RigidTransform(15).translation  TranslationROffset=0  TranslationROffsetUnits=m  TranslationZOffset=0  TranslationZOffsetUnits=m  TranslationThetaOffset=0  TranslationThetaOffsetUnits=deg  RotationMethod=ArbitraryAxis  RotationAngleUnits=rad  RotationStandardAxis=+Z  RotationAngle=smiData.RigidTransform(15).angle  RotationArbitraryAxis=smiData.RigidTransform(15).axis  FollAlignAxisA=+X  BaseAlignAxisA=+Y  FollAlignAxisB=+Y  BaseAlignAxisB=+Z  RotationSequenceAxes=FollowerAxes  RotationSequence=XYX  RotationSequenceAngles=[0 0 0]  RotationSequenceAnglesUnits=deg  RotationMatrix=[1 0 0; 0 1 0; 0 0 1]
  F1 : PMIOPort  Side=Left
  F : PMIOPort  Port=2  Side=Left
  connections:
  Solid/RConn1 -- ReferenceFrame/RConn1 -- Transform/LConn1 -- Transform1/LConn1
  Transform/RConn1 -- F/RConn1
  Transform1/RConn1 -- F1/RConn1

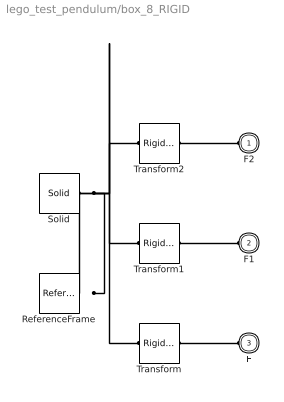
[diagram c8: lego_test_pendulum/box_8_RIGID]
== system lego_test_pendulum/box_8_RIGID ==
  ReferenceFrame : sm_lib/Frames and Transforms/Reference Frame
  Solid : sm_lib/Body Elements/Solid  InertiaType=Custom  Mass=smiData.Solid(1).mass  MassUnits=kg  CenterOfMass=smiData.Solid(1).CoM  CenterOfMassUnits=mm  MomentsOfInertia=smiData.Solid(1).MoI  MomentsOfInertiaUnits=kg*mm^2  ProductsOfInertia=smiData.Solid(1).PoI  ProductsOfInertiaUnits=kg*mm^2  DensityBased=on  Density=1000  DensityUnits=kg/m^3  DoExposeReferenceFrame=on  SerializedFrames=<Frames/>  GraphicType=FromGeometry  MarkerShape=Sphere  MarkerSize=10  GraphicVisPropType=SimpleVisualProperties  GraphicDiffuseColor=smiData.Solid(1).color  GraphicSpecularColor=[0.5 0.5 0.5 1.0]  GraphicAmbientColor=[0.15 0.15 0.15 1.0]  GraphicEmissiveColor=[0.0 0.0 0.0 1.0]  GraphicShininess=75  GraphicOpacity=smiData.Solid(1).opacity  GeometryShape=FromFile  RectangleSize=[1 1]  RectangleSizeUnits=m  BrickDimensions=[1 1 1]  BrickDimensionUnits=m  CylinderRadius=1  CylinderRadiusUnits=m  CylinderLength=1  CylinderLengthUnits=m  SphereRadius=1  SphereRadiusUnits=m  EllipsoidRadii=[1 1 1]  EllipsoidRadiiUnits=m  ExtrusionCrossSection=[1 1; -1 1; -1 -1; 1 -1]  ExtrusionCrossSectionUnits=m  ExtrusionLength=1  ExtrusionLengthUnits=m  PolygonNumSides=3  PolygonOuterRadius=1  PolygonOuterRadiusUnits=m  ExtGeomFileType=STEP  ExtGeomFileName=box_Predeterminado_sldprt.STEP  ExtGeomFileUnits=m  RevolutionCrossSection=[1 1; 1 -1; 2 -1; 2 1]  RevolutionCrossSectionUnits=m  RevolutionExtent=Full  RevolutionAngle=180  RevolutionAngleUnits=deg
  Transform : sm_lib/Frames and Transforms/Rigid Transform  TranslationMethod=Cartesian  TranslationStandardOffset=0  TranslationLengthUnit=mm  TranslationStandardAxis=+Z  TranslationCartesianOffset=smiData.RigidTransform(16).translation  TranslationROffset=0  TranslationROffsetUnits=m  TranslationZOffset=0  TranslationZOffsetUnits=m  TranslationThetaOffset=0  TranslationThetaOffsetUnits=deg  RotationMethod=ArbitraryAxis  RotationAngleUnits=rad  RotationStandardAxis=+Z  RotationAngle=smiData.RigidTransform(16).angle  RotationArbitraryAxis=smiData.RigidTransform(16).axis  FollAlignAxisA=+X  BaseAlignAxisA=+Y  FollAlignAxisB=+Y  BaseAlignAxisB=+Z  RotationSequenceAxes=FollowerAxes  RotationSequence=XYX  RotationSequenceAngles=[0 0 0]  RotationSequenceAnglesUnits=deg  RotationMatrix=[1 0 0; 0 1 0; 0 0 1]
  Transform1 : sm_lib/Frames and Transforms/Rigid Transform  TranslationMethod=Cartesian  TranslationStandardOffset=0  TranslationLengthUnit=mm  TranslationStandardAxis=+Z  TranslationCartesianOffset=smiData.RigidTransform(18).translation  TranslationROffset=0  TranslationROffsetUnits=m  TranslationZOffset=0  TranslationZOffsetUnits=m  TranslationThetaOffset=0  TranslationThetaOffsetUnits=deg  RotationMethod=ArbitraryAxis  RotationAngleUnits=rad  RotationStandardAxis=+Z  RotationAngle=smiData.RigidTransform(18).angle  RotationArbitraryAxis=smiData.RigidTransform(18).axis  FollAlignAxisA=+X  BaseAlignAxisA=+Y  FollAlignAxisB=+Y  BaseAlignAxisB=+Z  RotationSequenceAxes=FollowerAxes  RotationSequence=XYX  RotationSequenceAngles=[0 0 0]  RotationSequenceAnglesUnits=deg  RotationMatrix=[1 0 0; 0 1 0; 0 0 1]
  Transform2 : sm_lib/Frames and Transforms/Rigid Transform  TranslationMethod=Cartesian  TranslationStandardOffset=0  TranslationLengthUnit=mm  TranslationStandardAxis=+Z  TranslationCartesianOffset=smiData.RigidTransform(20).translation  TranslationROffset=0  TranslationROffsetUnits=m  TranslationZOffset=0  TranslationZOffsetUnits=m  TranslationThetaOffset=0  TranslationThetaOffsetUnits=deg  RotationMethod=ArbitraryAxis  RotationAngleUnits=rad  RotationStandardAxis=+Z  RotationAngle=smiData.RigidTransform(20).angle  RotationArbitraryAxis=smiData.RigidTransform(20).axis  FollAlignAxisA=+X  BaseAlignAxisA=+Y  FollAlignAxisB=+Y  BaseAlignAxisB=+Z  RotationSequenceAxes=FollowerAxes  RotationSequence=XYX  RotationSequenceAngles=[0 0 0]  RotationSequenceAnglesUnits=deg  RotationMatrix=[1 0 0; 0 1 0; 0 0 1]
  F2 : PMIOPort  Side=Left
  F1 : PMIOPort  Port=2  Side=Left
  F : PMIOPort  Port=3  Side=Left
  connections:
  Solid/RConn1 -- ReferenceFrame/RConn1 -- Transform/LConn1 -- Transform1/LConn1 -- Transform2/LConn1
  Transform/RConn1 -- F/RConn1
  Transform1/RConn1 -- F1/RConn1
  Transform2/RConn1 -- F2/RConn1

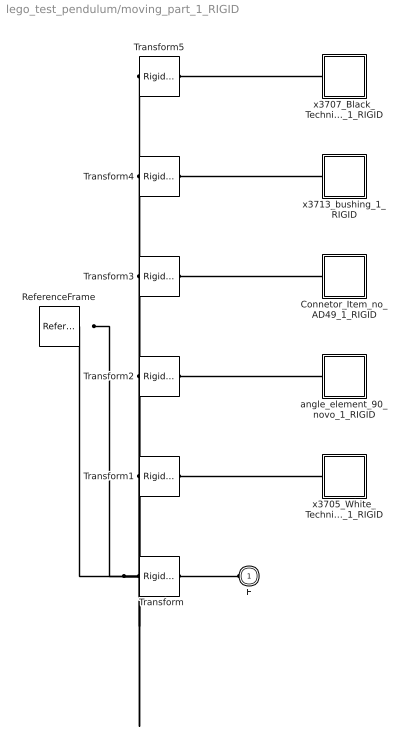
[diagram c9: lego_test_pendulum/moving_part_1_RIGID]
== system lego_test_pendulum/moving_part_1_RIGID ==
  Connetor_Item_no_AD49_1_RIGID : Subsystem
  ReferenceFrame : sm_lib/Frames and Transforms/Reference Frame
  Transform : sm_lib/Frames and Transforms/Rigid Transform  TranslationMethod=Cartesian  TranslationStandardOffset=0  TranslationLengthUnit=mm  TranslationStandardAxis=+Z  TranslationCartesianOffset=smiData.RigidTransform(2).translation  TranslationROffset=0  TranslationROffsetUnits=m  TranslationZOffset=0  TranslationZOffsetUnits=m  TranslationThetaOffset=0  TranslationThetaOffsetUnits=deg  RotationMethod=ArbitraryAxis  RotationAngleUnits=rad  RotationStandardAxis=+Z  RotationAngle=smiData.RigidTransform(2).angle  RotationArbitraryAxis=smiData.RigidTransform(2).axis  FollAlignAxisA=+X  BaseAlignAxisA=+Y  FollAlignAxisB=+Y  BaseAlignAxisB=+Z  RotationSequenceAxes=FollowerAxes  RotationSequence=XYX  RotationSequenceAngles=[0 0 0]  RotationSequenceAnglesUnits=deg  RotationMatrix=[1 0 0; 0 1 0; 0 0 1]
  Transform1 : sm_lib/Frames and Transforms/Rigid Transform  TranslationMethod=Cartesian  TranslationStandardOffset=0  TranslationLengthUnit=mm  TranslationStandardAxis=+Z  TranslationCartesianOffset=smiData.RigidTransform(21).translation  TranslationROffset=0  TranslationROffsetUnits=m  TranslationZOffset=0  TranslationZOffsetUnits=m  TranslationThetaOffset=0  TranslationThetaOffsetUnits=deg  RotationMethod=ArbitraryAxis  RotationAngleUnits=rad  RotationStandardAxis=+Z  RotationAngle=smiData.RigidTransform(21).angle  RotationArbitraryAxis=smiData.RigidTransform(21).axis  FollAlignAxisA=+X  BaseAlignAxisA=+Y  FollAlignAxisB=+Y  BaseAlignAxisB=+Z  RotationSequenceAxes=FollowerAxes  RotationSequence=XYX  RotationSequenceAngles=[0 0 0]  RotationSequenceAnglesUnits=deg  RotationMatrix=[1 0 0; 0 1 0; 0 0 1]
  Transform2 : sm_lib/Frames and Transforms/Rigid Transform  TranslationMethod=Cartesian  TranslationStandardOffset=0  TranslationLengthUnit=mm  TranslationStandardAxis=+Z  TranslationCartesianOffset=smiData.RigidTransform(22).translation  TranslationROffset=0  TranslationROffsetUnits=m  TranslationZOffset=0  TranslationZOffsetUnits=m  TranslationThetaOffset=0  TranslationThetaOffsetUnits=deg  RotationMethod=ArbitraryAxis  RotationAngleUnits=rad  RotationStandardAxis=+Z  RotationAngle=smiData.RigidTransform(22).angle  RotationArbitraryAxis=smiData.RigidTransform(22).axis  FollAlignAxisA=+X  BaseAlignAxisA=+Y  FollAlignAxisB=+Y  BaseAlignAxisB=+Z  RotationSequenceAxes=FollowerAxes  RotationSequence=XYX  RotationSequenceAngles=[0 0 0]  RotationSequenceAnglesUnits=deg  RotationMatrix=[1 0 0; 0 1 0; 0 0 1]
  Transform3 : sm_lib/Frames and Transforms/Rigid Transform  TranslationMethod=Cartesian  TranslationStandardOffset=0  TranslationLengthUnit=mm  TranslationStandardAxis=+Z  TranslationCartesianOffset=smiData.RigidTransform(23).translation  TranslationROffset=0  TranslationROffsetUnits=m  TranslationZOffset=0  TranslationZOffsetUnits=m  TranslationThetaOffset=0  TranslationThetaOffsetUnits=deg  RotationMethod=ArbitraryAxis  RotationAngleUnits=rad  RotationStandardAxis=+Z  RotationAngle=smiData.RigidTransform(23).angle  RotationArbitraryAxis=smiData.RigidTransform(23).axis  FollAlignAxisA=+X  BaseAlignAxisA=+Y  FollAlignAxisB=+Y  BaseAlignAxisB=+Z  RotationSequenceAxes=FollowerAxes  RotationSequence=XYX  RotationSequenceAngles=[0 0 0]  RotationSequenceAnglesUnits=deg  RotationMatrix=[1 0 0; 0 1 0; 0 0 1]
  Transform4 : sm_lib/Frames and Transforms/Rigid Transform  TranslationMethod=Cartesian  TranslationStandardOffset=0  TranslationLengthUnit=mm  TranslationStandardAxis=+Z  TranslationCartesianOffset=smiData.RigidTransform(24).translation  TranslationROffset=0  TranslationROffsetUnits=m  TranslationZOffset=0  TranslationZOffsetUnits=m  TranslationThetaOffset=0  TranslationThetaOffsetUnits=deg  RotationMethod=ArbitraryAxis  RotationAngleUnits=rad  RotationStandardAxis=+Z  RotationAngle=smiData.RigidTransform(24).angle  RotationArbitraryAxis=smiData.RigidTransform(24).axis  FollAlignAxisA=+X  BaseAlignAxisA=+Y  FollAlignAxisB=+Y  BaseAlignAxisB=+Z  RotationSequenceAxes=FollowerAxes  RotationSequence=XYX  RotationSequenceAngles=[0 0 0]  RotationSequenceAnglesUnits=deg  RotationMatrix=[1 0 0; 0 1 0; 0 0 1]
  Transform5 : sm_lib/Frames and Transforms/Rigid Transform  TranslationMethod=Cartesian  TranslationStandardOffset=0  TranslationLengthUnit=mm  TranslationStandardAxis=+Z  TranslationCartesianOffset=smiData.RigidTransform(25).translation  TranslationROffset=0  TranslationROffsetUnits=m  TranslationZOffset=0  TranslationZOffsetUnits=m  TranslationThetaOffset=0  TranslationThetaOffsetUnits=deg  RotationMethod=ArbitraryAxis  RotationAngleUnits=rad  RotationStandardAxis=+Z  RotationAngle=smiData.RigidTransform(25).angle  RotationArbitraryAxis=smiData.RigidTransform(25).axis  FollAlignAxisA=+X  BaseAlignAxisA=+Y  FollAlignAxisB=+Y  BaseAlignAxisB=+Z  RotationSequenceAxes=FollowerAxes  RotationSequence=XYX  RotationSequenceAngles=[0 0 0]  RotationSequenceAnglesUnits=deg  RotationMatrix=[1 0 0; 0 1 0; 0 0 1]
  angle_element_90_novo_1_RIGID : Subsystem
  x3705_White_Technic_Axle_4_1_RIGID : Subsystem
  x3707_Black_Technic_Axle_8_1_RIGID : Subsystem
  x3713_bushing_1_RIGID : Subsystem
  F : PMIOPort  Side=Left
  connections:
  Transform/LConn1 -- ReferenceFrame/RConn1 -- Transform1/LConn1 -- Transform2/LConn1 -- Transform3/LConn1 -- Transform4/LConn1 -- Transform5/LConn1
  Transform/RConn1 -- F/RConn1
  Transform1/RConn1 -- x3705_White_Technic_Axle_4_1_RIGID/LConn1
  Transform2/RConn1 -- angle_element_90_novo_1_RIGID/LConn1
  Connetor_Item_no_AD49_1_RIGID/LConn1 -- Transform3/RConn1
  Transform4/RConn1 -- x3713_bushing_1_RIGID/LConn1
  Transform5/RConn1 -- x3707_Black_Technic_Axle_8_1_RIGID/LConn1

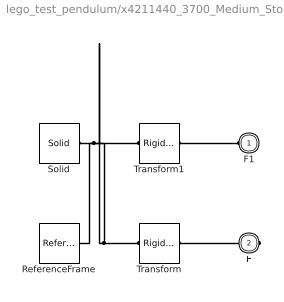
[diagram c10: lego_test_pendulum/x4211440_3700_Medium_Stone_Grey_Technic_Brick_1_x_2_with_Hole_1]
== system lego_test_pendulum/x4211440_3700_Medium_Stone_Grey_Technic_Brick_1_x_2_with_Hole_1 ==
  ReferenceFrame : sm_lib/Frames and Transforms/Reference Frame
  Solid : sm_lib/Body Elements/Solid  InertiaType=Custom  Mass=smiData.Solid(7).mass  MassUnits=kg  CenterOfMass=smiData.Solid(7).CoM  CenterOfMassUnits=mm  MomentsOfInertia=smiData.Solid(7).MoI  MomentsOfInertiaUnits=kg*mm^2  ProductsOfInertia=smiData.Solid(7).PoI  ProductsOfInertiaUnits=kg*mm^2  DensityBased=on  Density=1000  DensityUnits=kg/m^3  DoExposeReferenceFrame=on  SerializedFrames=<Frames/>  GraphicType=FromGeometry  MarkerShape=Sphere  MarkerSize=10  GraphicVisPropType=SimpleVisualProperties  GraphicDiffuseColor=smiData.Solid(7).color  GraphicSpecularColor=[0.5 0.5 0.5 1.0]  GraphicAmbientColor=[0.15 0.15 0.15 1.0]  GraphicEmissiveColor=[0.0 0.0 0.0 1.0]  GraphicShininess=75  GraphicOpacity=smiData.Solid(7).opacity  GeometryShape=FromFile  RectangleSize=[1 1]  RectangleSizeUnits=m  BrickDimensions=[1 1 1]  BrickDimensionUnits=m  CylinderRadius=1  CylinderRadiusUnits=m  CylinderLength=1  CylinderLengthUnits=m  SphereRadius=1  SphereRadiusUnits=m  EllipsoidRadii=[1 1 1]  EllipsoidRadiiUnits=m  ExtrusionCrossSection=[1 1; -1 1; -1 -1; 1 -1]  ExtrusionCrossSectionUnits=m  ExtrusionLength=1  ExtrusionLengthUnits=m  PolygonNumSides=3  PolygonOuterRadius=1  PolygonOuterRadiusUnits=m  ExtGeomFileType=STEP  ExtGeomFileName=4211440 - 3700 Medium Stone Grey Technic Brick 1 x 2 with Hole_Predeterminado_sldprt.STEP  ExtGeomFileUnits=m  RevolutionCrossSection=[1 1; 1 -1; 2 -1; 2 1]  RevolutionCrossSectionUnits=m  RevolutionExtent=Full  RevolutionAngle=180  RevolutionAngleUnits=deg
  Transform : sm_lib/Frames and Transforms/Rigid Transform  TranslationMethod=Cartesian  TranslationStandardOffset=0  TranslationLengthUnit=mm  TranslationStandardAxis=+Z  TranslationCartesianOffset=smiData.RigidTransform(1).translation  TranslationROffset=0  TranslationROffsetUnits=m  TranslationZOffset=0  TranslationZOffsetUnits=m  TranslationThetaOffset=0  TranslationThetaOffsetUnits=deg  RotationMethod=ArbitraryAxis  RotationAngleUnits=rad  RotationStandardAxis=+Z  RotationAngle=smiData.RigidTransform(1).angle  RotationArbitraryAxis=smiData.RigidTransform(1).axis  FollAlignAxisA=+X  BaseAlignAxisA=+Y  FollAlignAxisB=+Y  BaseAlignAxisB=+Z  RotationSequenceAxes=FollowerAxes  RotationSequence=XYX  RotationSequenceAngles=[0 0 0]  RotationSequenceAnglesUnits=deg  RotationMatrix=[1 0 0; 0 1 0; 0 0 1]
  Transform1 : sm_lib/Frames and Transforms/Rigid Transform  TranslationMethod=Cartesian  TranslationStandardOffset=0  TranslationLengthUnit=mm  TranslationStandardAxis=+Z  TranslationCartesianOffset=smiData.RigidTransform(17).translation  TranslationROffset=0  TranslationROffsetUnits=m  TranslationZOffset=0  TranslationZOffsetUnits=m  TranslationThetaOffset=0  TranslationThetaOffsetUnits=deg  RotationMethod=ArbitraryAxis  RotationAngleUnits=rad  RotationStandardAxis=+Z  RotationAngle=smiData.RigidTransform(17).angle  RotationArbitraryAxis=smiData.RigidTransform(17).axis  FollAlignAxisA=+X  BaseAlignAxisA=+Y  FollAlignAxisB=+Y  BaseAlignAxisB=+Z  RotationSequenceAxes=FollowerAxes  RotationSequence=XYX  RotationSequenceAngles=[0 0 0]  RotationSequenceAnglesUnits=deg  RotationMatrix=[1 0 0; 0 1 0; 0 0 1]
  F1 : PMIOPort  Side=Left
  F : PMIOPort  Port=2  Side=Right
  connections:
  Solid/RConn1 -- ReferenceFrame/RConn1 -- Transform/LConn1 -- Transform1/LConn1
  Transform/RConn1 -- F/RConn1
  Transform1/RConn1 -- F1/RConn1

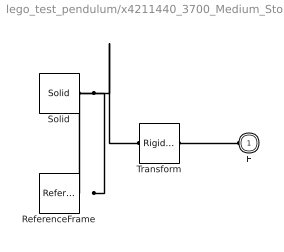
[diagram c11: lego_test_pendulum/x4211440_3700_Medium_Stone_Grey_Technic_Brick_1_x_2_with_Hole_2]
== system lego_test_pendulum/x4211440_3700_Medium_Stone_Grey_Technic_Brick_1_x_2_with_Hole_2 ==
  ReferenceFrame : sm_lib/Frames and Transforms/Reference Frame
  Solid : sm_lib/Body Elements/Solid  InertiaType=Custom  Mass=smiData.Solid(7).mass  MassUnits=kg  CenterOfMass=smiData.Solid(7).CoM  CenterOfMassUnits=mm  MomentsOfInertia=smiData.Solid(7).MoI  MomentsOfInertiaUnits=kg*mm^2  ProductsOfInertia=smiData.Solid(7).PoI  ProductsOfInertiaUnits=kg*mm^2  DensityBased=on  Density=1000  DensityUnits=kg/m^3  DoExposeReferenceFrame=on  SerializedFrames=<Frames/>  GraphicType=FromGeometry  MarkerShape=Sphere  MarkerSize=10  GraphicVisPropType=SimpleVisualProperties  GraphicDiffuseColor=smiData.Solid(7).color  GraphicSpecularColor=[0.5 0.5 0.5 1.0]  GraphicAmbientColor=[0.15 0.15 0.15 1.0]  GraphicEmissiveColor=[0.0 0.0 0.0 1.0]  GraphicShininess=75  GraphicOpacity=smiData.Solid(7).opacity  GeometryShape=FromFile  RectangleSize=[1 1]  RectangleSizeUnits=m  BrickDimensions=[1 1 1]  BrickDimensionUnits=m  CylinderRadius=1  CylinderRadiusUnits=m  CylinderLength=1  CylinderLengthUnits=m  SphereRadius=1  SphereRadiusUnits=m  EllipsoidRadii=[1 1 1]  EllipsoidRadiiUnits=m  ExtrusionCrossSection=[1 1; -1 1; -1 -1; 1 -1]  ExtrusionCrossSectionUnits=m  ExtrusionLength=1  ExtrusionLengthUnits=m  PolygonNumSides=3  PolygonOuterRadius=1  PolygonOuterRadiusUnits=m  ExtGeomFileType=STEP  ExtGeomFileName=4211440 - 3700 Medium Stone Grey Technic Brick 1 x 2 with Hole_Predeterminado_sldprt.STEP  ExtGeomFileUnits=m  RevolutionCrossSection=[1 1; 1 -1; 2 -1; 2 1]  RevolutionCrossSectionUnits=m  RevolutionExtent=Full  RevolutionAngle=180  RevolutionAngleUnits=deg
  Transform : sm_lib/Frames and Transforms/Rigid Transform  TranslationMethod=Cartesian  TranslationStandardOffset=0  TranslationLengthUnit=mm  TranslationStandardAxis=+Z  TranslationCartesianOffset=smiData.RigidTransform(19).translation  TranslationROffset=0  TranslationROffsetUnits=m  TranslationZOffset=0  TranslationZOffsetUnits=m  TranslationThetaOffset=0  TranslationThetaOffsetUnits=deg  RotationMethod=ArbitraryAxis  RotationAngleUnits=rad  RotationStandardAxis=+Z  RotationAngle=smiData.RigidTransform(19).angle  RotationArbitraryAxis=smiData.RigidTransform(19).axis  FollAlignAxisA=+X  BaseAlignAxisA=+Y  FollAlignAxisB=+Y  BaseAlignAxisB=+Z  RotationSequenceAxes=FollowerAxes  RotationSequence=XYX  RotationSequenceAngles=[0 0 0]  RotationSequenceAnglesUnits=deg  RotationMatrix=[1 0 0; 0 1 0; 0 0 1]
  F : PMIOPort  Side=Left
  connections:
  Solid/RConn1 -- ReferenceFrame/RConn1 -- Transform/LConn1
  Transform/RConn1 -- F/RConn1

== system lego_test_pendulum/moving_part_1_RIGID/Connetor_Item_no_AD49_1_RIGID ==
  ReferenceFrame : sm_lib/Frames and Transforms/Reference Frame
  Solid : sm_lib/Body Elements/Solid  InertiaType=Custom  Mass=smiData.Solid(4).mass  MassUnits=kg  CenterOfMass=smiData.Solid(4).CoM  CenterOfMassUnits=mm  MomentsOfInertia=smiData.Solid(4).MoI  MomentsOfInertiaUnits=kg*mm^2  ProductsOfInertia=smiData.Solid(4).PoI  ProductsOfInertiaUnits=kg*mm^2  DensityBased=on  Density=1000  DensityUnits=kg/m^3  DoExposeReferenceFrame=on  SerializedFrames=<Frames/>  GraphicType=FromGeometry  MarkerShape=Sphere  MarkerSize=10  GraphicVisPropType=SimpleVisualProperties  GraphicDiffuseColor=smiData.Solid(4).color  GraphicSpecularColor=[0.5 0.5 0.5 1.0]  GraphicAmbientColor=[0.15 0.15 0.15 1.0]  GraphicEmissiveColor=[0.0 0.0 0.0 1.0]  GraphicShininess=75  GraphicOpacity=smiData.Solid(4).opacity  GeometryShape=FromFile  RectangleSize=[1 1]  RectangleSizeUnits=m  BrickDimensions=[1 1 1]  BrickDimensionUnits=m  CylinderRadius=1  CylinderRadiusUnits=m  CylinderLength=1  CylinderLengthUnits=m  SphereRadius=1  SphereRadiusUnits=m  EllipsoidRadii=[1 1 1]  EllipsoidRadiiUnits=m  ExtrusionCrossSection=[1 1; -1 1; -1 -1; 1 -1]  ExtrusionCrossSectionUnits=m  ExtrusionLength=1  ExtrusionLengthUnits=m  PolygonNumSides=3  PolygonOuterRadius=1  PolygonOuterRadiusUnits=m  ExtGeomFileType=STEP  ExtGeomFileName=Connetor - Item no AD49_Default_sldprt.STEP  ExtGeomFileUnits=m  RevolutionCrossSection=[1 1; 1 -1; 2 -1; 2 1]  RevolutionCrossSectionUnits=m  RevolutionExtent=Full  RevolutionAngle=180  RevolutionAngleUnits=deg
  F : PMIOPort  Side=Left
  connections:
  Solid/RConn1 -- ReferenceFrame/RConn1 -- F/RConn1

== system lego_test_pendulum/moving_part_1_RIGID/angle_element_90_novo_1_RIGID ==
  ReferenceFrame : sm_lib/Frames and Transforms/Reference Frame
  Solid : sm_lib/Body Elements/Solid  InertiaType=Custom  Mass=smiData.Solid(3).mass  MassUnits=kg  CenterOfMass=smiData.Solid(3).CoM  CenterOfMassUnits=mm  MomentsOfInertia=smiData.Solid(3).MoI  MomentsOfInertiaUnits=kg*mm^2  ProductsOfInertia=smiData.Solid(3).PoI  ProductsOfInertiaUnits=kg*mm^2  DensityBased=on  Density=1000  DensityUnits=kg/m^3  DoExposeReferenceFrame=on  SerializedFrames=<Frames/>  GraphicType=FromGeometry  MarkerShape=Sphere  MarkerSize=10  GraphicVisPropType=SimpleVisualProperties  GraphicDiffuseColor=smiData.Solid(3).color  GraphicSpecularColor=[0.5 0.5 0.5 1.0]  GraphicAmbientColor=[0.15 0.15 0.15 1.0]  GraphicEmissiveColor=[0.0 0.0 0.0 1.0]  GraphicShininess=75  GraphicOpacity=smiData.Solid(3).opacity  GeometryShape=FromFile  RectangleSize=[1 1]  RectangleSizeUnits=m  BrickDimensions=[1 1 1]  BrickDimensionUnits=m  CylinderRadius=1  CylinderRadiusUnits=m  CylinderLength=1  CylinderLengthUnits=m  SphereRadius=1  SphereRadiusUnits=m  EllipsoidRadii=[1 1 1]  EllipsoidRadiiUnits=m  ExtrusionCrossSection=[1 1; -1 1; -1 -1; 1 -1]  ExtrusionCrossSectionUnits=m  ExtrusionLength=1  ExtrusionLengthUnits=m  PolygonNumSides=3  PolygonOuterRadius=1  PolygonOuterRadiusUnits=m  ExtGeomFileType=STEP  ExtGeomFileName=angle element 90 novo_Default_sldprt.STEP  ExtGeomFileUnits=m  RevolutionCrossSection=[1 1; 1 -1; 2 -1; 2 1]  RevolutionCrossSectionUnits=m  RevolutionExtent=Full  RevolutionAngle=180  RevolutionAngleUnits=deg
  F : PMIOPort  Side=Left
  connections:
  Solid/RConn1 -- ReferenceFrame/RConn1 -- F/RConn1
